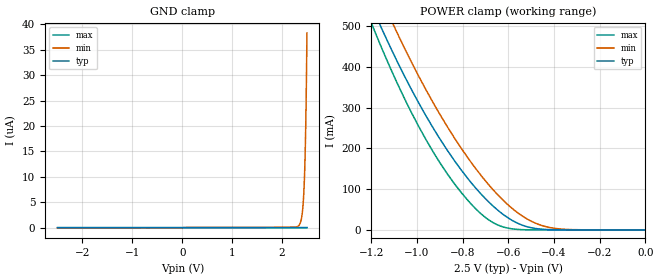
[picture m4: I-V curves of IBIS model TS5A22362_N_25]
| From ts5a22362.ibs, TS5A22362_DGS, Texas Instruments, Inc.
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[Model]   TS5A22362_N_25
Model_type  Terminator
| variable   typ   min   max
C_comp   70.48pF   66.83pF   75.67pF
| C_tri-state   70.48pF   66.83pF   75.67pF
[Temperature Range]   40   100   -40
| Ambient temperature   25   85   -40
[Voltage range]   2.5   2.3   2.7
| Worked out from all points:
|   POWER clamp passes 1 mA (typ) near -0.43 V on its own axis
[GND Clamp]
| TS5A22362_N_25
|   Voltage   I(typ)   I(min)   I(max)
-2.5V     -933.4pA   -100.3nA   -148.5pA
2.325V    619.6pA    316.6nA    22.3pA
2.365V    630.6pA    884.1nA    23.45pA
2.395V    645pA      2.054uA    24.31pA
2.42V     670.5pA    4.185uA    25.03pA
2.44V     713.6pA    7.373uA    25.6pA
2.45V     750.2pA    9.761uA    25.88pA
2.46V     803.4pA    12.9uA     26.17pA
2.475V    933pA      19.49uA    26.59pA
2.485V    1.072nA    25.59uA    26.88pA
2.49V     1.164nA    29.29uA    27.02pA
2.5V      1.412nA    38.3uA     27.3pA
[POWER Clamp]
| TS5A22362_N_25
|   Voltage   I(typ)   I(min)   I(max)
-2.5V     3.132A     3.191A     3.415A
-1.195V   546.1mA    619.7mA    502.4mA
-1.18V    527mA      600.1mA    481.7mA
-1.145V   483.3mA    555.4mA    434.7mA
-1.085V   412.3mA    482.1mA    359.1mA
-930mV    251.5mA    313.6mA    192.9mA
-805mV    146.5mA    199.8mA    91.31mA
-690mV    71.21mA    113.8mA    26.49mA
-570mV    19.47mA    46.93mA    1.916mA
-480mV    3.559mA    16.43mA    107.1uA
-395mV    430.1uA    3.782mA    4.223uA
0V        0A         0A         0A
